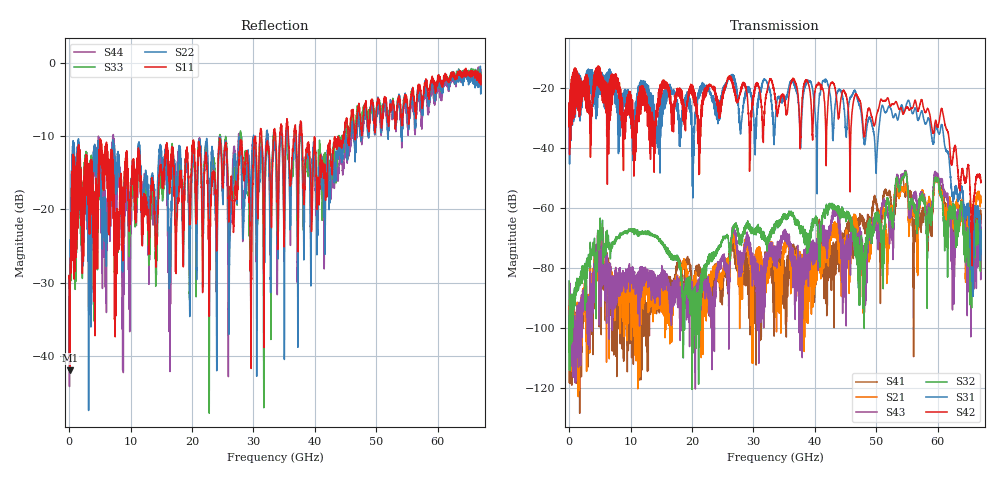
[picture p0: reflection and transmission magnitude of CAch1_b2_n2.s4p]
!Agilent Technologies,N5247A,US51170199,A.09.90.13
!Agilent N5247A: A.09.90.13
!Date: Thursday, October 18, 2018 09:18:25
!Correction: S11(Full 4 Port(1,2,3,4))
!S12(Full 4 Port(1,2,3,4))
!S13(Full 4 Port(1,2,3,4))
!S14(Full 4 Port(1,2,3,4))
!S21(Full 4 Port(1,2,3,4))
!S22(Full 4 Port(1,2,3,4))
!S23(Full 4 Port(1,2,3,4))
!S24(Full 4 Port(1,2,3,4))
!S31(Full 4 Port(1,2,3,4))
!S32(Full 4 Port(1,2,3,4))
!S33(Full 4 Port(1,2,3,4))
!S34(Full 4 Port(1,2,3,4))
!S41(Full 4 Port(1,2,3,4))
!S42(Full 4 Port(1,2,3,4))
!S43(Full 4 Port(1,2,3,4))
!S44(Full 4 Port(1,2,3,4))
!S4P File: Measurements: <S11,S12,S13,S14>,
!<S21,S22,S23,S24>,
!<S31,S32,S33,S34>,
!<S41,S42,S43,S44>:
# Hz S  dB  R 50
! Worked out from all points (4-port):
!   6701 points, 10 MHz to 67 GHz, reference 50 ohm
!   strongest paths, dB at 10 MHz, 16.76 GHz, 33.51 GHz, 50.25 GHz, 67 GHz:
!     S42: -32.7, -32.0, -23.6, -27.5, -51.1
!     S31: -32.9, -22.0, -32.6, -37.1, -68.4
!     S32: -84.3, -76.8, -66.1, -61.5, -67.3
!     S43: -97.0, -92.3, -75.9, -68.9, -75.9
!     S21: -90.8, -90.1, -79.6, -64.1, -57.6
!     S41: -97.1, -86.4, -87.6, -62.5, -62.1
!   lowest |S11| = -41.9 dB at 140 MHz (marker M1), VSWR 1.02, Z = 50 - j0.799 ohm
!   |S11| at or under -10 dB: start of sweep to 31.04 GHz; 31.34 GHz to 33.31 GHz (1.975 GHz wide, 6.11 % of centre); 37.9 GHz to 44.54 GHz (6.635 GHz wide, 16.1 % of centre)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
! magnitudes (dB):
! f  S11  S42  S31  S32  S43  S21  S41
! 10 MHz  -29.4  -32.7  -32.9  -84.3  -97.0  -90.8  -97.1
! 140 MHz  -41.9  -24.9  -24.5  -96.0  -97.4  -93.1  -95.8
! 42.65 GHz  -13.8  -18.3  -25.8  -58.6  -64.0  -69.4  -77.6
! 47.84 GHz  -7.8  -33.0  -34.8  -93.6  -73.5  -92.8  -65.0
! 55.19 GHz  -6.7  -26.7  -24.0  -55.6  -57.0  -60.1  -54.1
! 65.6 GHz  -1.1  -79.3  -71.0  -84.8  -77.3  -61.1  -68.7
! 67 GHz  -3.0  -51.1  -68.4  -67.3  -75.9  -57.6  -62.1
